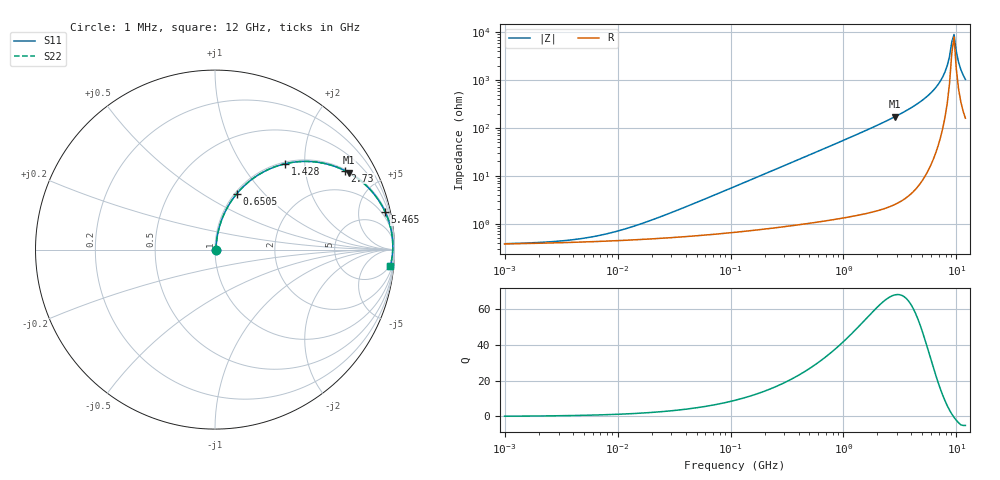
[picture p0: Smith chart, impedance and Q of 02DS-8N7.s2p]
# MHz S MA R 50
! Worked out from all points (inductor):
!   204 points, 1 MHz to 12 GHz, reference 50 ohm
!   read as one part in series: L = 8.7 nH near 27.98 MHz
!   highest Q = 67.9 at 2.859 GHz (marker M1), where L = 9.59 nH
!   self-resonance near 9.091 GHz
!   S11 on the Smith chart (normalised r, x): 1 MHz: 1.01, +0.00; 650.5 MHz: 1.02, +0.71; 1.428 GHz: 1.03, +1.60; 2.73 GHz: 1.05, +3.26; 5.465 GHz: 1.23, +9.02; 12 GHz: 4, -20
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1  0.003825 8.2  0.9962 -0.0  0.9962 -0.0  0.003825 8.2
4.82184  0.004903 32.2  0.9959 -0.2  0.9959 -0.2  0.004903 32.2
10.1094  0.007066 50.8  0.9956 -0.3  0.9956 -0.3  0.007066 50.8
23.2501  0.01357 68.0  0.995 -0.7  0.995 -0.7  0.01357 68.0
112.108  0.06113 80.3  0.9915 -3.5  0.9915 -3.5  0.06113 80.3
257.833  0.1388 78.7  0.9822 -8.0  0.9822 -8.0  0.1388 78.7
540.568  0.2817 71.6  0.9496 -16.4  0.9496 -16.4  0.2817 71.6
650.472  0.3333 68.7  0.9324 -19.5  0.9324 -19.5  0.3333 68.7
1428.35  0.6186 50.7  0.7738 -38.2  0.7738 -38.2  0.6186 50.7
2606.53  0.8336 32.7  0.54 -56.5  0.54 -56.5  0.8336 32.7
2729.97  0.8468 31.3  0.5195 -57.9  0.5195 -57.9  0.8468 31.3
2859.25  0.8594 29.9  0.4989 -59.2  0.4989 -59.2  0.8594 29.9
4140.07  0.9372 19.5  0.3337 -69.6  0.3337 -69.6  0.9372 19.5
5464.81  0.9711 12.4  0.2152 -76.1  0.2152 -76.1  0.9711 12.4
6887.27  0.9862 7.0  0.1214 -80.0  0.1214 -80.0  0.9862 7.0
7912.81  0.9902 3.8  0.06711 -79.7  0.06711 -79.7  0.9902 3.8
8680  0.9909 1.8  0.03198 -72.6  0.03198 -72.6  0.9909 1.8
9091.06  0.9907 0.7  0.0159 -53.8  0.0159 -53.8  0.9907 0.7
9521.58  0.9901 -0.3  0.01105 25.7  0.01105 25.7  0.9901 -0.3
9972.48  0.989 -1.3  0.02502 63.4  0.02502 63.4  0.989 -1.3
10444.7  0.9876 -2.3  0.042 71.7  0.042 71.7  0.9876 -2.3
12000  0.9809 -5.4  0.09487 75.7  0.09487 75.7  0.9809 -5.4
